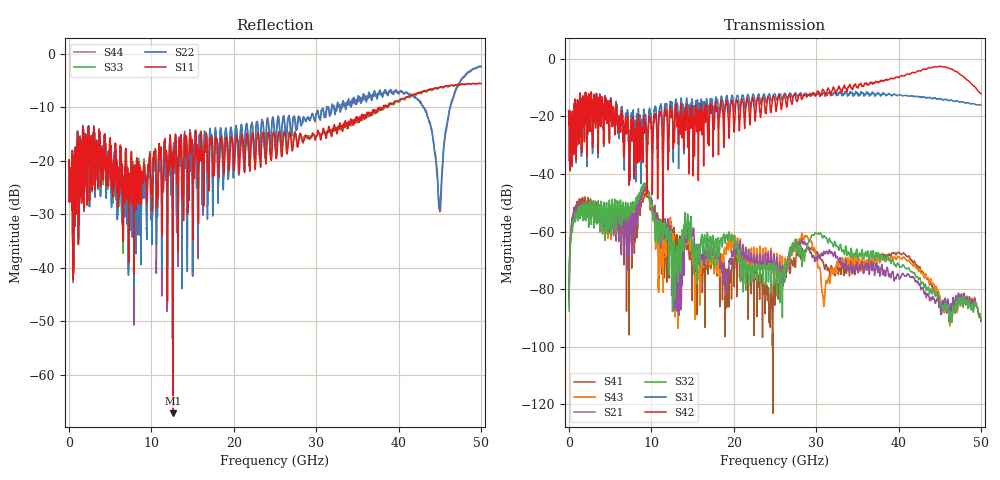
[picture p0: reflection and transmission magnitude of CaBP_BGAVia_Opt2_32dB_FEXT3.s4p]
!* Samtec Inc. NovaRay Examax Flyover System  *
!*  REV DATE  = 08/08/18  *
!*  TYPE  = TOUCHSTONE  *
!*  PORTS  = 4 port  *
!*  UNITS  = GHz  *
!*  DATA RANGE = DC  to 50 GHz; 10 MHz Step  *
!*  PARAMETER  = S  *
!*  FORMAT  = Real-Imaginary  *
!*  REFERENCE  = 50 ohms  *
!*  SOURCE  = HFSS  *
!*  VALIDATED  = No  *
!*  MANUFACTURER = SAMTEC  *
!*  INTERCONNECT = NVAx to EBCx to EBCx to NVAx  *
!*  [Full Channel NVAx to EBCx to EBCx to NVAx  with PCB Trace and BGA Via]  *
!*  BOUNDARY A  = Silicon BGA Ball Pad  *
!*  BOUNDARY B  = Silicon BGA Ball Pad  *
!*  NVAx (end a) ->>- (end b) NVAx  *
!*  Port 01 ->>- Port 02  *
!*  Port 03 ->>- Port 04  *
!***************************** CHANNEL MODEL ******************************************
# GHz S RI R 50
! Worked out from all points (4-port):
!   5000 points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, 10 MHz to 50 GHz, reference 50 ohm
!   strongest paths, dB at 10 MHz, 12.51 GHz, 25.01 GHz, 37.51 GHz, 50 GHz:
!     S42: -23.1, -18.2, -14.7, -8.2, -12.1
!     S31: -23.1, -15.2, -12.2, -11.7, -16.1
!     S32: -87.7, -71.5, -72.0, -68.9, -90.5
!     S21: -85.2, -66.1, -72.5, -74.1, -91.2
!     S43: -85.8, -61.9, -74.3, -69.4, -90.7
!     S41: -83.6, -61.4, -81.9, -68.5, -91.2
!   lowest |S11| = -67.2 dB at 12.6 GHz (marker M1), VSWR 1.00, Z = 50 + j0.0147 ohm
!   |S11| at or under -10 dB: start of sweep to 37.74 GHz; 37.74 GHz to 38.13 GHz (385.5 MHz wide, 1.02 % of centre); 38.51568 GHz to 38.54961 GHz (33.93 MHz wide, 0.0881 % of centre)
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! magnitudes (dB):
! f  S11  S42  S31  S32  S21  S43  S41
! 10 MHz  -21.6  -23.1  -23.1  -87.7  -85.2  -85.8  -83.6
! 1.09 GHz  -17.6  -18.2  -18.3  -53.3  -51.8  -52.2  -50.8
! 9.21 GHz  -22.2  -24.7  -21.3  -43.7  -44.8  -45.5  -46.3
! 12.6 GHz  -67.2  -25.2  -21.8  -69.1  -67.1  -63.2  -62.8
! 40.2 GHz  -8.5  -6.1  -12.5  -72.3  -76.1  -69.0  -67.6
! 45.02 GHz  -6.3  -2.6  -13.9  -84.2  -85.1  -82.6  -83.8
! 50 GHz  -5.5  -12.1  -16.1  -90.5  -91.2  -90.7  -91.2
